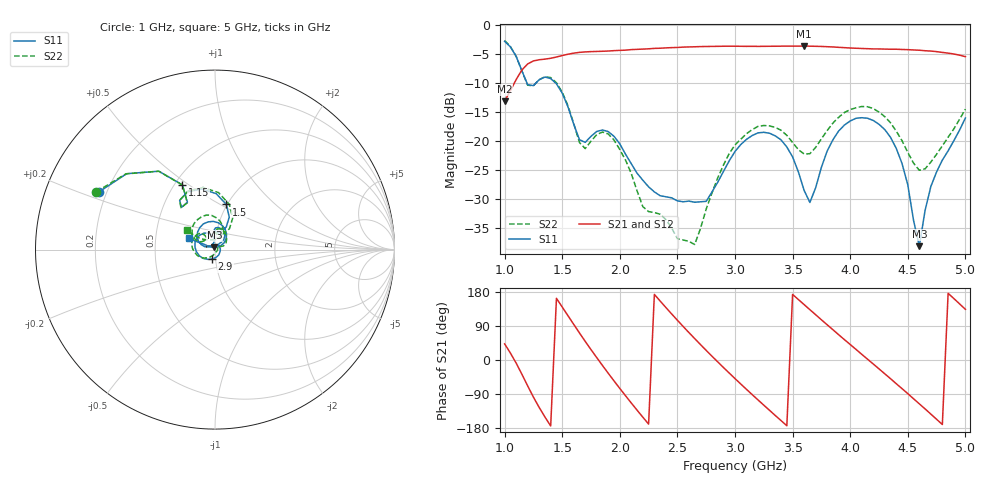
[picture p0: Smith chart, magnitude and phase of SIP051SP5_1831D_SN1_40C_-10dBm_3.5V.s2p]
# GHz  S  dB  R  50
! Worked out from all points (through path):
!   81 points, 1 GHz to 5 GHz, reference 50 ohm
!   highest |S21| = -3.64 dB at 3.6 GHz (marker M1); lowest = -13.1 dB at 1 GHz (marker M2)
!   lowest |S11| = -38.1 dB at 4.6 GHz (marker M3), VSWR 1.03, Z = 49.6 + j1.19 ohm
!   |S11| at or under -10 dB: 1.194 GHz to 1.272 GHz (77.97 MHz wide, 6.32 % of centre); 1.443 GHz to end of sweep
!   |S22| runs from -37.8 to -2.7 dB; largest |S21 - S12| = 0.0028
!   S11 on the Smith chart (normalised r, x): 1 GHz: 0.17, +0.23; 1.15 GHz: 0.55, +0.47; 1.5 GHz: 0.99, +0.53; 2.9 GHz: 0.96, -0.10; 5 GHz: 0.74, +0.10
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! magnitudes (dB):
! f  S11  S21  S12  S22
! 1 GHz  -2.8  -13.1  -13.1  -2.7
! 1.15 GHz  -7.9  -7.8  -7.8  -7.9
! 1.5 GHz  -11.7  -5.3  -5.3  -11.6
! 1.7 GHz  -20.2  -4.6  -4.6  -21.3
! 1.9 GHz  -18.4  -4.5  -4.5  -18.8
! 2.2 GHz  -26.7  -4.2  -4.2  -31.3
! 2.35 GHz  -29.4  -4.0  -4.0  -32.6
! 2.65 GHz  -30.5  -3.8  -3.8  -37.8
! 2.9 GHz  -25.2  -3.7  -3.7  -24.1
! 3 GHz  -21.8  -3.7  -3.7  -20.7
! 3.35 GHz  -19.1  -3.7  -3.7  -17.6
! 3.5 GHz  -22.7  -3.7  -3.6  -20.2
! 3.6 GHz  -28.5  -3.6  -3.7  -22.2
! 3.65 GHz  -30.6  -3.7  -3.7  -22.2
! 3.7 GHz  -28.0  -3.7  -3.7  -21.1
! 3.85 GHz  -19.8  -3.8  -3.8  -16.9
! 4 GHz  -16.5  -4.0  -4.0  -14.6
! 4.35 GHz  -19.3  -4.2  -4.2  -16.8
! 4.5 GHz  -27.5  -4.3  -4.2  -21.9
! 4.6 GHz  -38.1  -4.4  -4.4  -25.0
! 4.7 GHz  -27.8  -4.5  -4.5  -23.6
! 5 GHz  -16.0  -5.5  -5.5  -14.5
